(* Logix 5000 AddOnInstructionDefinition export Banner_K50ProL2_Param_v4; software revision 32.00 *)

TYPE Banner_IOL_Port_v4 :   // UDT that has all of the data items necessary to communicate with a specific Port on a IO-Link Master
STRUCT
   Port_Controlled : INT;   // Each bit represents a port on an IO-Link Master. Set to 1 to tell AOI to control that port.
   Port_Activate : INT;   // Each bit represents a port on an IO-Link Master. When ON that port will process any commands in queue.
   Port_Read : INT;   // Each bit represents a port on an IO-Link Master. Used to determine when device AOI has requested a Read command.
   Port_Write : INT;   // Each bit represents a port on an IO-Link Master. Used to determine when device AOI has requested a Write command.
   Port_RW_Complete : INT;   // Each bit represents a port on an IO-Link Master. Tells device AOI that Read or Write request has been completed.
   Port_Device_Read : INT;
   Data_Transfer : SINT[190];   // Array to transfer data from IO-Master to device AOIs.
END_STRUCT
END_TYPE

TYPE Banner_K50ProL2_CC_v2 :   // K50 Pro L2 Custom Color Setup Structure.
STRUCT
   Blue : INT;
   Green : INT;
   Red : INT;
   Color_Name : STRING;
END_STRUCT
END_TYPE

TYPE Banner_K50ProL2_RD_v2 :   // All of the read parameters for a K50 Pro L2
STRUCT
   Master_Cycle_Time : INT;
   Min_Cycle_Time : INT;
   M_Sequence_Capability : INT;
   IO_Link_Version_ID : INT;
   Process_Data_Input_Length : INT;
   Process_Data_Output_Length : INT;
   Combined_Vendor_ID : DINT;   // IO-Link Vendor ID
   Vendor_ID1 : INT;
   Vendor_ID2 : INT;
   Combined_Device_ID : DINT;   // IO-Link Device ID
   Device_ID1 : INT;
   Device_ID2 : INT;
   Device_ID3 : INT;
   Serial_Number : STRING;
END_STRUCT
END_TYPE

TYPE Banner_K50ProL2_v2 :   // All of the parameters for a K50 Pro L2.
STRUCT
   Initial_Global_Read : BOOL;   // Determines if all of the IO-Link data has been read into the PLC yet
   Command : INT;   // Value placed in here will activate a read or write to a specifc IO-Link Index
   Reset : BOOL;   // Resets AOI. This will force a complete parameter read of the sensor.
   Read_Data : Banner_K50ProL2_RD_v2;
   Write_Data : Banner_K50ProL2_WD_v2;
   Archive_Data : Banner_K50ProL2_WD_v2;
END_STRUCT
END_TYPE

TYPE Banner_K50ProL2_WD_v2 :   // All of the write parameters for a K50 Pro L2.
STRUCT
   System_Command : INT;
   Parameter_Access_Lock : SINT;
   Data_Storage_Lock : SINT;
   Local_Parameterization_Lock : SINT;
   Local_User_Interface_Lock : SINT;
   Reserved : INT;
   Restrict_To_Gamut : INT;
   Rotation_Speed : INT;
   Custom_Flash_Rate : INT;   // .5 to 20 Hz
   Custom_Intensity : INT;   // 0 to 100 = 0 to 100%
   Custom_Color : Banner_K50ProL2_CC_v2[6];
END_STRUCT
END_TYPE

ADD_ON_INSTRUCTION Banner_K50ProL2_Param_v4   (* revision 4.0, vendor Banner Engineering *)
// AOI to read and write parameter data to an IO-Link K50 Pro L2.
VAR_IN_OUT
   K50ProL2 : Banner_K50ProL2_v2; {required}
   Port_Data : Banner_IOL_Port_v4; {required}
END_VAR
VAR_INPUT
   Port : DINT; {required}
END_VAR
VAR
   Local_Control : DINT; {access None}
   Global_Read_Command_Value : INT; {access None}
   Global_Write_Command_Value : INT; {access None}
   Command_Being_Processed : BOOL; {access None}
   Index_Write_Inprocess : INT; {access None}
   Index_Write_Control : INT; {access None}
   Update_Archive : BOOL; {access None}
   Inprocess_Index : DINT; {access None}
   CC_R_Index : DINT; {access None}
   CC_WC_Index : DINT; {access None}
   CC_Index : DINT; {access None}
   CC_W_Index : DINT; {access None}
   CC_WC2_Index : DINT; {access None}
END_VAR

ROUTINE Logic   (* ladder *)
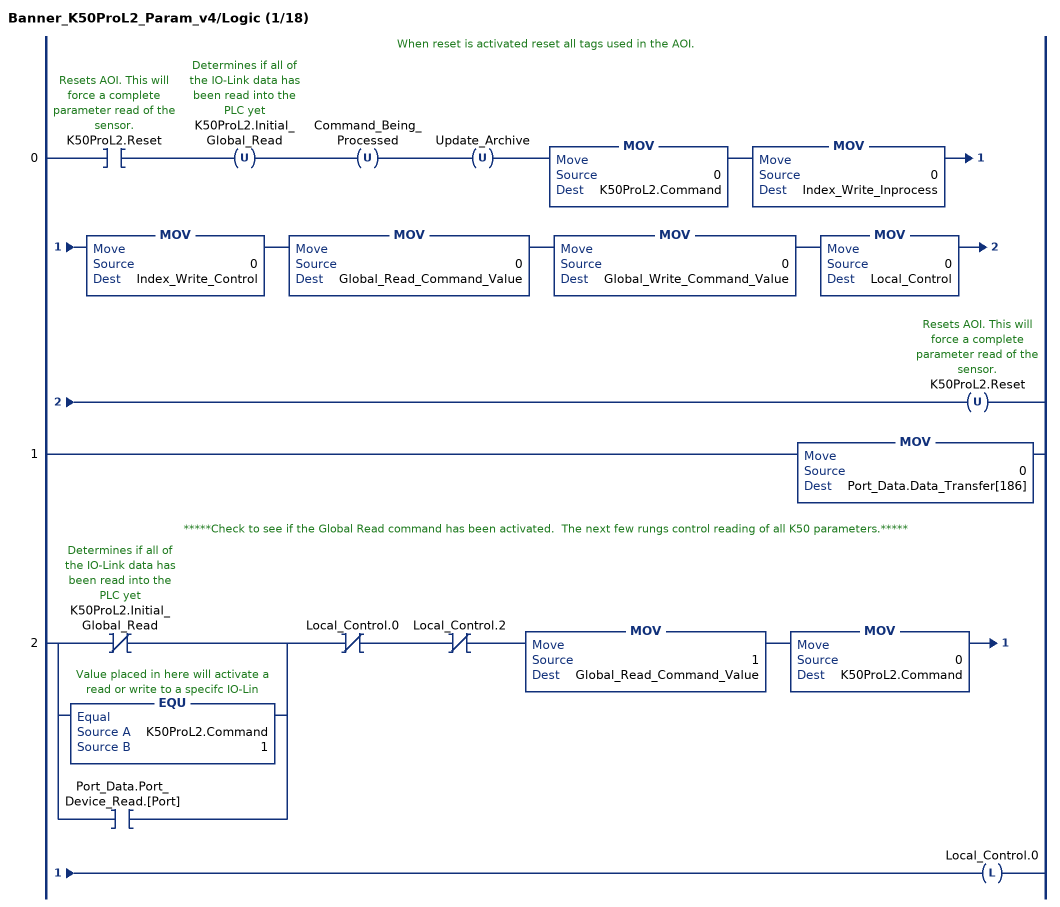
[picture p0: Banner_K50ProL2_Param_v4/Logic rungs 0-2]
   // When reset is activated reset all tags used in the AOI.
   0: XIC(K50ProL2.Reset)OTU(K50ProL2.Initial_Global_Read)OTU(Command_Being_Processed)OTU(Update_Archive)MOV(0,K50ProL2.Command)MOV(0,Index_Write_Inprocess)MOV(0,Index_Write_Control)MOV(0,Global_Read_Command_Value)MOV(0,Global_Write_Command_Value)MOV(0,Local_Control)OTU(K50ProL2.Reset);
   1: MOV(0,Port_Data.Data_Transfer[186]);
   // *****Check to see if the Global Read command has been activated.  The next few rungs control reading of all K50 parameters.*****
   2: [XIO(K50ProL2.Initial_Global_Read) ,EQU(K50ProL2.Command,1) ,XIC(Port_Data.Port_Device_Read.[Port]) ]XIO(Local_Control.0)XIO(Local_Control.2)MOV(1,Global_Read_Command_Value)MOV(0,K50ProL2.Command)OTL(Local_Control.0);
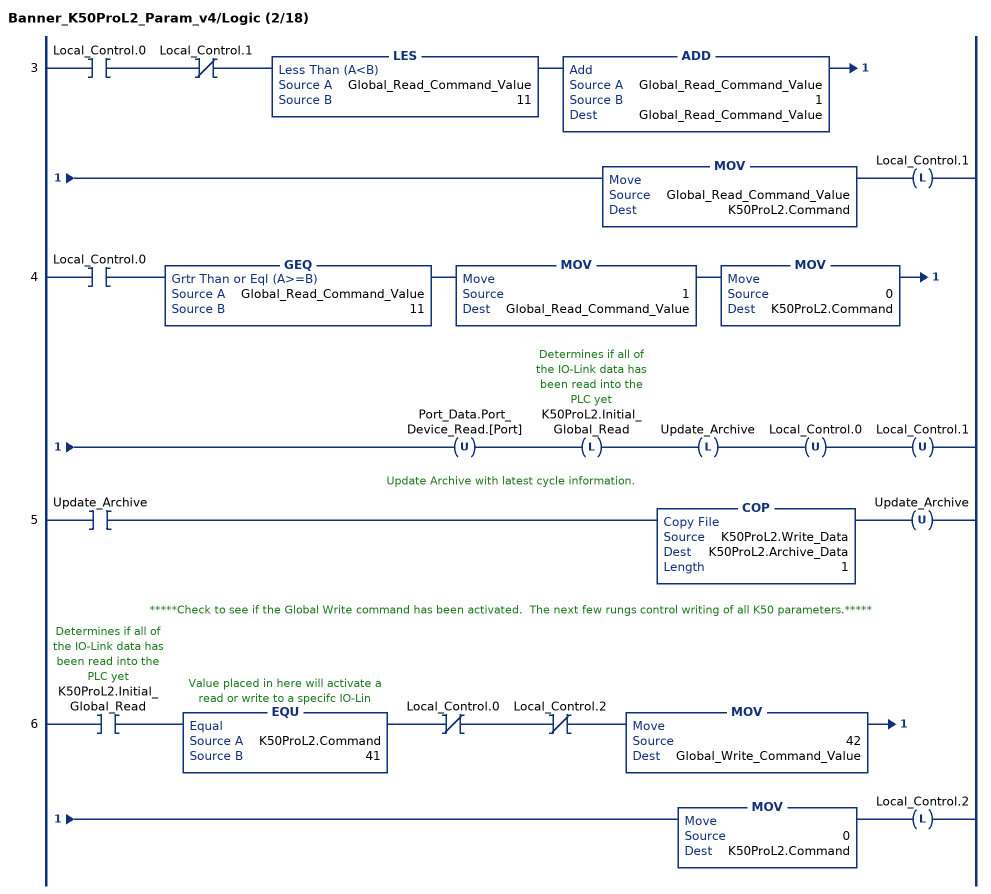
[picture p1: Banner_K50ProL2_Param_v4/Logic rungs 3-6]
   3: XIC(Local_Control.0)XIO(Local_Control.1)LES(Global_Read_Command_Value,11)ADD(Global_Read_Command_Value,1,Global_Read_Command_Value)MOV(Global_Read_Command_Value,K50ProL2.Command)OTL(Local_Control.1);
   4: XIC(Local_Control.0)GEQ(Global_Read_Command_Value,11)MOV(1,Global_Read_Command_Value)MOV(0,K50ProL2.Command)OTU(Port_Data.Port_Device_Read.[Port])OTL(K50ProL2.Initial_Global_Read)OTL(Update_Archive)OTU(Local_Control.0)OTU(Local_Control.1);
   // Update Archive with latest cycle information.
   5: XIC(Update_Archive)COP(K50ProL2.Write_Data,K50ProL2.Archive_Data,1)OTU(Update_Archive);
   // *****Check to see if the Global Write command has been activated.  The next few rungs control writing of all K50 parameters.*****
   6: XIC(K50ProL2.Initial_Global_Read)EQU(K50ProL2.Command,41)XIO(Local_Control.0)XIO(Local_Control.2)MOV(42,Global_Write_Command_Value)MOV(0,K50ProL2.Command)OTL(Local_Control.2);
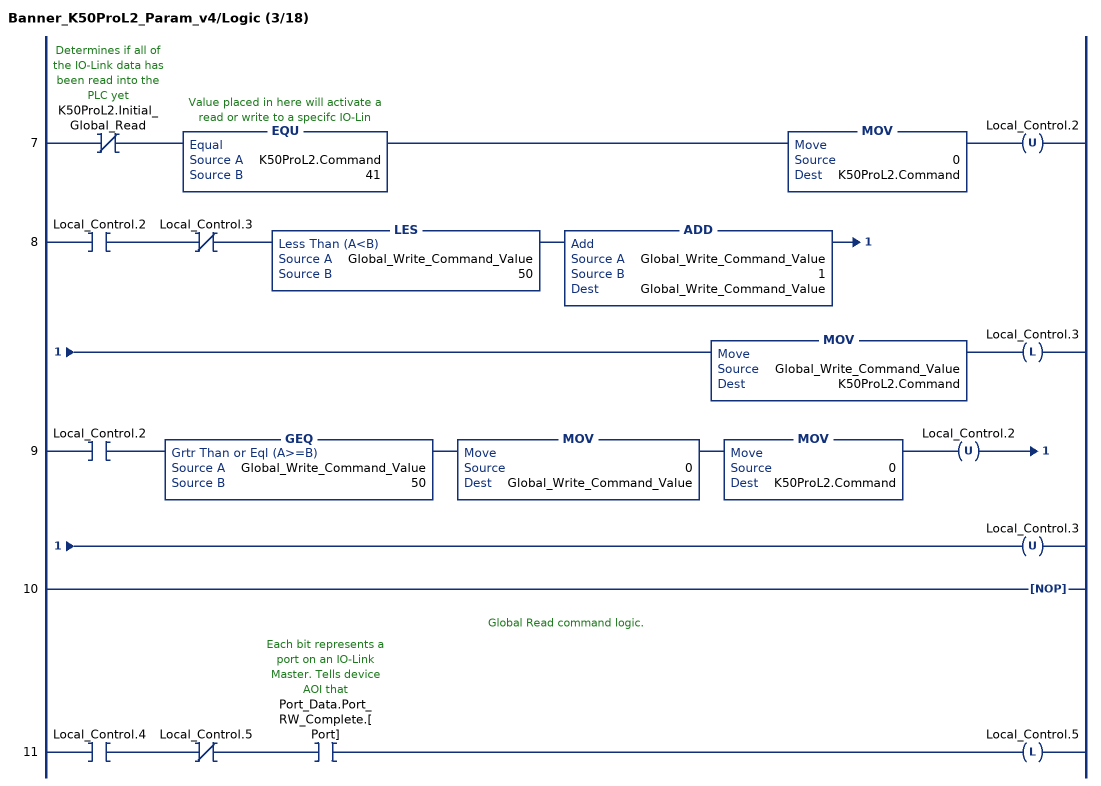
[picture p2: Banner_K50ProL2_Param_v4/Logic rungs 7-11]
   7: XIO(K50ProL2.Initial_Global_Read)EQU(K50ProL2.Command,41)MOV(0,K50ProL2.Command)OTU(Local_Control.2);
   8: XIC(Local_Control.2)XIO(Local_Control.3)LES(Global_Write_Command_Value,50)ADD(Global_Write_Command_Value,1,Global_Write_Command_Value)MOV(Global_Write_Command_Value,K50ProL2.Command)OTL(Local_Control.3);
   9: XIC(Local_Control.2)GEQ(Global_Write_Command_Value,50)MOV(0,Global_Write_Command_Value)MOV(0,K50ProL2.Command)OTU(Local_Control.2)OTU(Local_Control.3);
   10: NOP();
   // Global Read command logic.
   11: XIC(Local_Control.4)XIO(Local_Control.5)XIC(Port_Data.Port_RW_Complete.[Port])OTL(Local_Control.5);
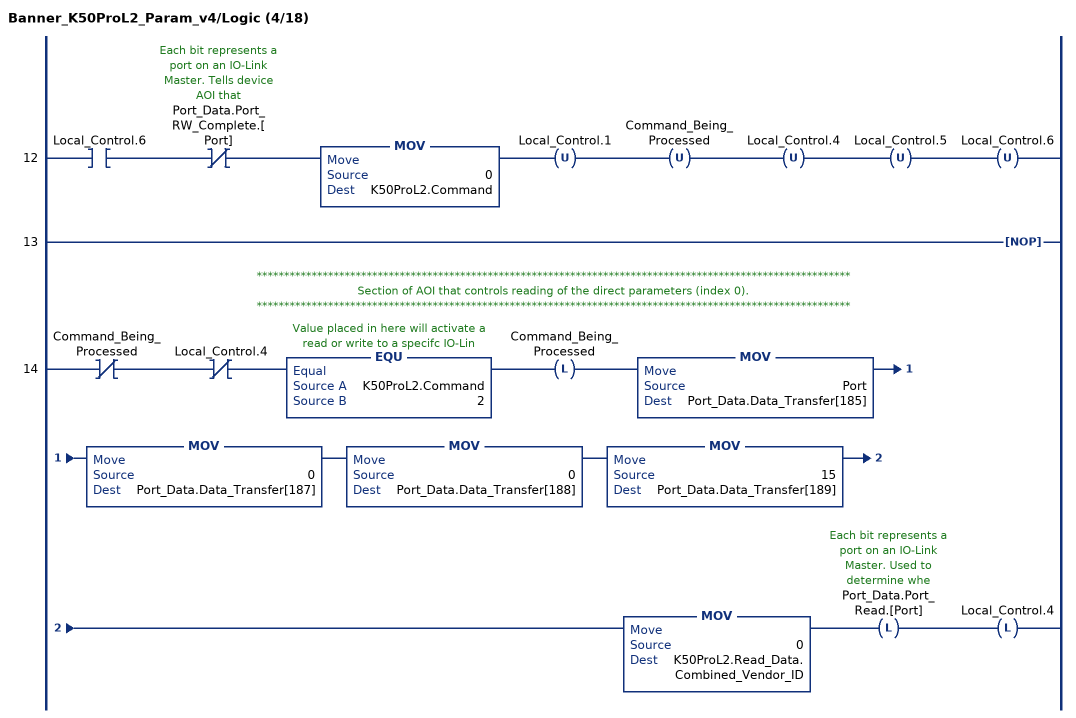
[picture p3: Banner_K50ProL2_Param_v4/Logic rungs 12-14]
   12: XIC(Local_Control.6)XIO(Port_Data.Port_RW_Complete.[Port])MOV(0,K50ProL2.Command)OTU(Local_Control.1)OTU(Command_Being_Processed)OTU(Local_Control.4)OTU(Local_Control.5)OTU(Local_Control.6);
   13: NOP();
   // ************************************************************************************************************
   // Section of AOI that controls reading of the direct parameters (index 0).
   // ************************************************************************************************************
   14: XIO(Command_Being_Processed)XIO(Local_Control.4)EQU(K50ProL2.Command,2)OTL(Command_Being_Processed)MOV(Port,Port_Data.Data_Transfer[185])MOV(0,Port_Data.Data_Transfer[187])MOV(0,Port_Data.Data_Transfer[188])MOV(15,Port_Data.Data_Transfer[189])MOV(0,K50ProL2.Read_Data.Combined_Vendor_ID)OTL(Port_Data.Port_Read.[Port])OTL(Local_Control.4);
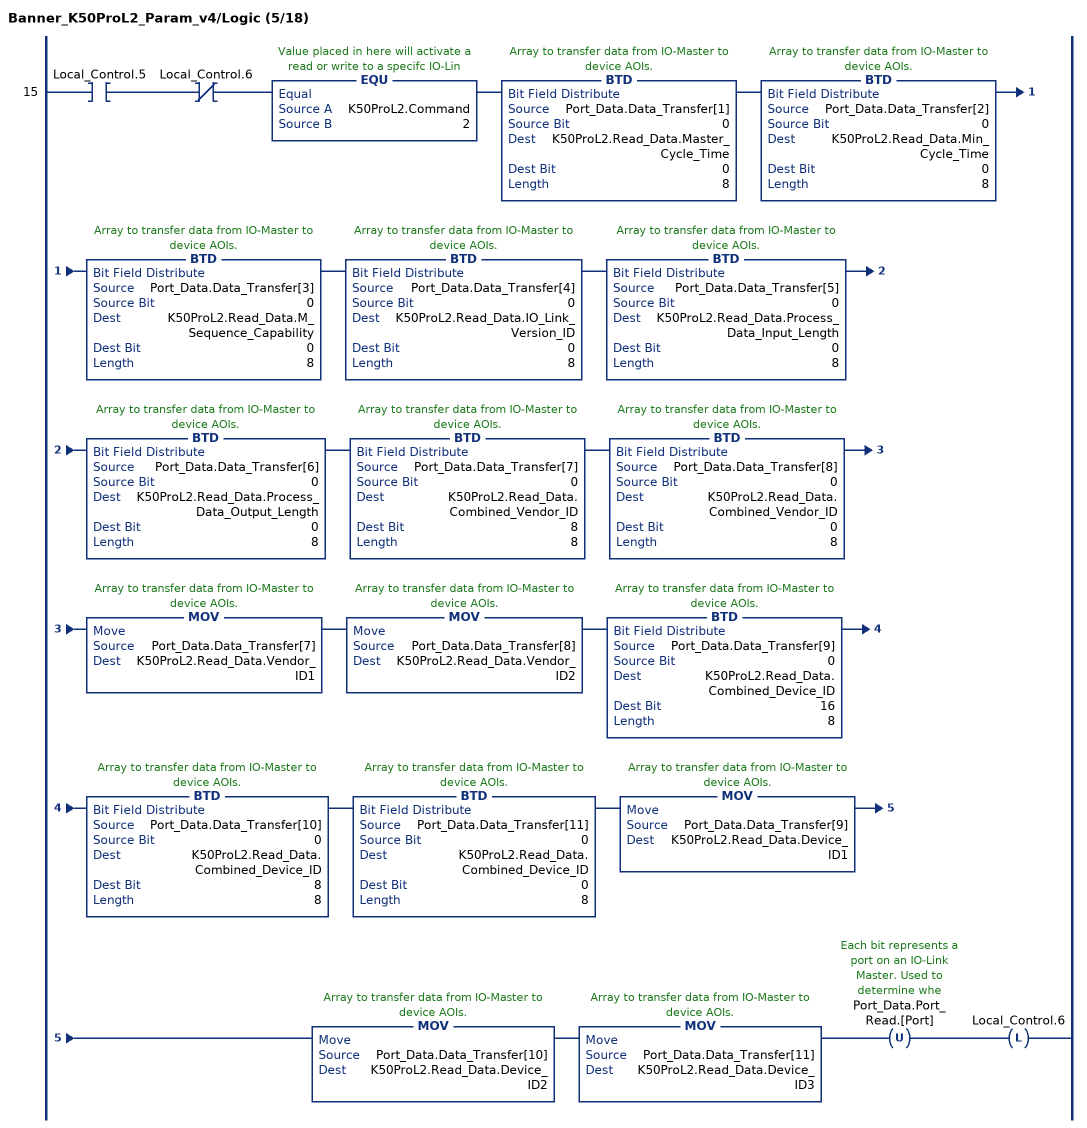
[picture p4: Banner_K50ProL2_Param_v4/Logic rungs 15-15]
   15: XIC(Local_Control.5)XIO(Local_Control.6)EQU(K50ProL2.Command,2)BTD(Port_Data.Data_Transfer[1],0,K50ProL2.Read_Data.Master_Cycle_Time,0,8)BTD(Port_Data.Data_Transfer[2],0,K50ProL2.Read_Data.Min_Cycle_Time,0,8)BTD(Port_Data.Data_Transfer[3],0,K50ProL2.Read_Data.M_Sequence_Capability,0,8)BTD(Port_Data.Data_Transfer[4],0,K50ProL2.Read_Data.IO_Link_Version_ID,0,8)BTD(Port_Data.Data_Transfer[5],0,K50ProL2.Read_Data.Process_Data_Input_Length,0,8)BTD(Port_Data.Data_Transfer[6],0,K50ProL2.Read_Data.Process_Data_Output_Length,0,8)BTD(Port_Data.Data_Transfer[7],0,K50ProL2.Read_Data.Combined_Vendor_ID,8,8)BTD(Port_Data.Data_Transfer[8],0,K50ProL2.Read_Data.Combined_Vendor_ID,0,8)MOV(Port_Data.Data_Transfer[7],K50ProL2.Read_Data.Vendor_ID1)MOV(Port_Data.Data_Transfer[8],K50ProL2.Read_Data.Vendor_ID2)BTD(Port_Data.Data_Transfer[9],0,K50ProL2.Read_Data.Combined_Device_ID,16,8)BTD(Port_Data.Data_Transfer[10],0,K50ProL2.Read_Data.Combined_Device_ID,8,8)BTD(Port_Data.Data_Transfer[11],0,K50ProL2.Read_Data.Combined_Device_ID,0,8)MOV(Port_Data.Data_Transfer[9],K50ProL2.Read_Data.Device_ID1)MOV(Port_Data.Data_Transfer[10],K50ProL2.Read_Data.Device_ID2)MOV(Port_Data.Data_Transfer[11],K50ProL2.Read_Data.Device_ID3)OTU(Port_Data.Port_Read.[Port])OTL(Local_Control.6);
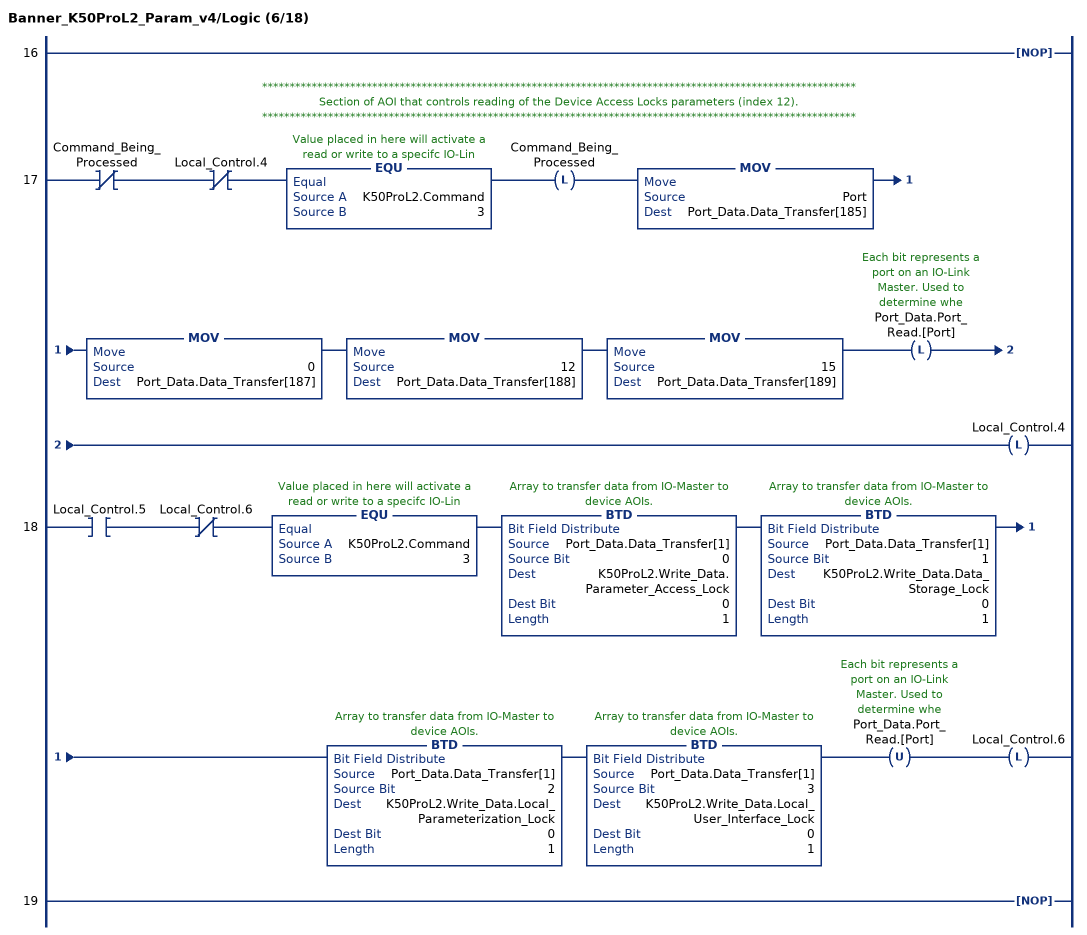
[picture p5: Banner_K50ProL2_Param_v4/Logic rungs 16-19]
   16: NOP();
   // ************************************************************************************************************
   // Section of AOI that controls reading of the Device Access Locks parameters (index 12).
   // ************************************************************************************************************
   17: XIO(Command_Being_Processed)XIO(Local_Control.4)EQU(K50ProL2.Command,3)OTL(Command_Being_Processed)MOV(Port,Port_Data.Data_Transfer[185])MOV(0,Port_Data.Data_Transfer[187])MOV(12,Port_Data.Data_Transfer[188])MOV(15,Port_Data.Data_Transfer[189])OTL(Port_Data.Port_Read.[Port])OTL(Local_Control.4);
   18: XIC(Local_Control.5)XIO(Local_Control.6)EQU(K50ProL2.Command,3)BTD(Port_Data.Data_Transfer[1],0,K50ProL2.Write_Data.Parameter_Access_Lock,0,1)BTD(Port_Data.Data_Transfer[1],1,K50ProL2.Write_Data.Data_Storage_Lock,0,1)BTD(Port_Data.Data_Transfer[1],2,K50ProL2.Write_Data.Local_Parameterization_Lock,0,1)BTD(Port_Data.Data_Transfer[1],3,K50ProL2.Write_Data.Local_User_Interface_Lock,0,1)OTU(Port_Data.Port_Read.[Port])OTL(Local_Control.6);
   19: NOP();
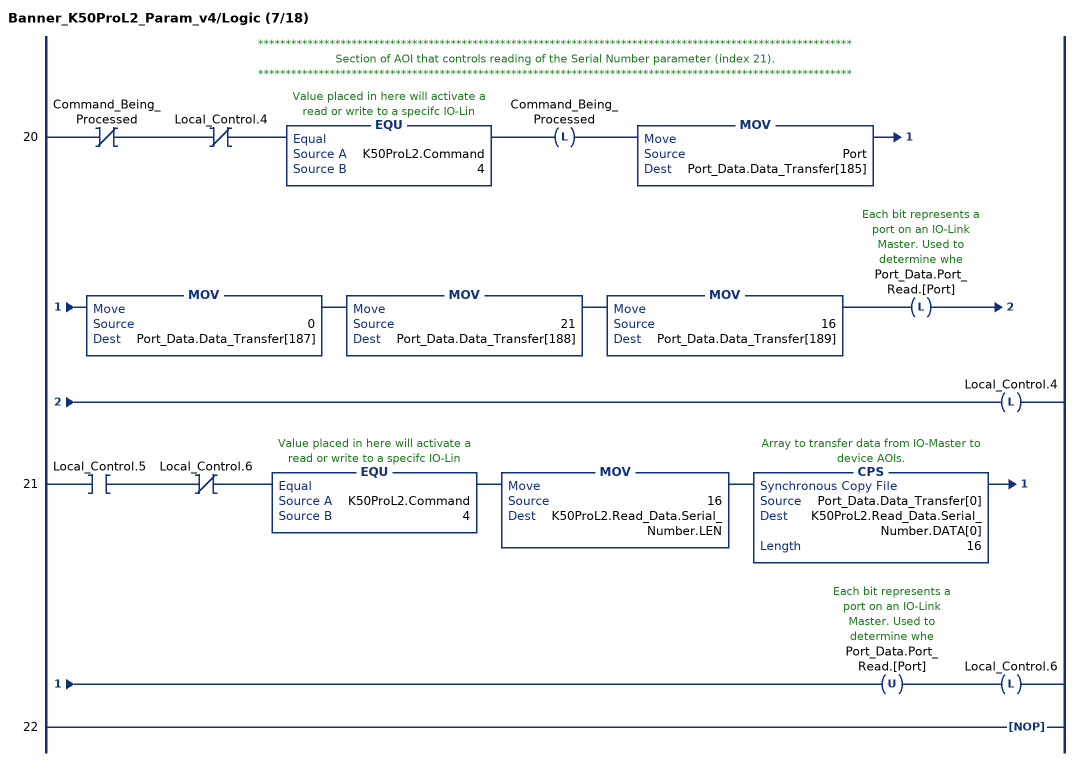
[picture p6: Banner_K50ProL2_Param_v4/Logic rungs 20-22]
   // ************************************************************************************************************
   // Section of AOI that controls reading of the Serial Number parameter (index 21).
   // ************************************************************************************************************
   20: XIO(Command_Being_Processed)XIO(Local_Control.4)EQU(K50ProL2.Command,4)OTL(Command_Being_Processed)MOV(Port,Port_Data.Data_Transfer[185])MOV(0,Port_Data.Data_Transfer[187])MOV(21,Port_Data.Data_Transfer[188])MOV(16,Port_Data.Data_Transfer[189])OTL(Port_Data.Port_Read.[Port])OTL(Local_Control.4);
   21: XIC(Local_Control.5)XIO(Local_Control.6)EQU(K50ProL2.Command,4)MOV(16,K50ProL2.Read_Data.Serial_Number.LEN)CPS(Port_Data.Data_Transfer[0],K50ProL2.Read_Data.Serial_Number.DATA[0],16)OTU(Port_Data.Port_Read.[Port])OTL(Local_Control.6);
   22: NOP();
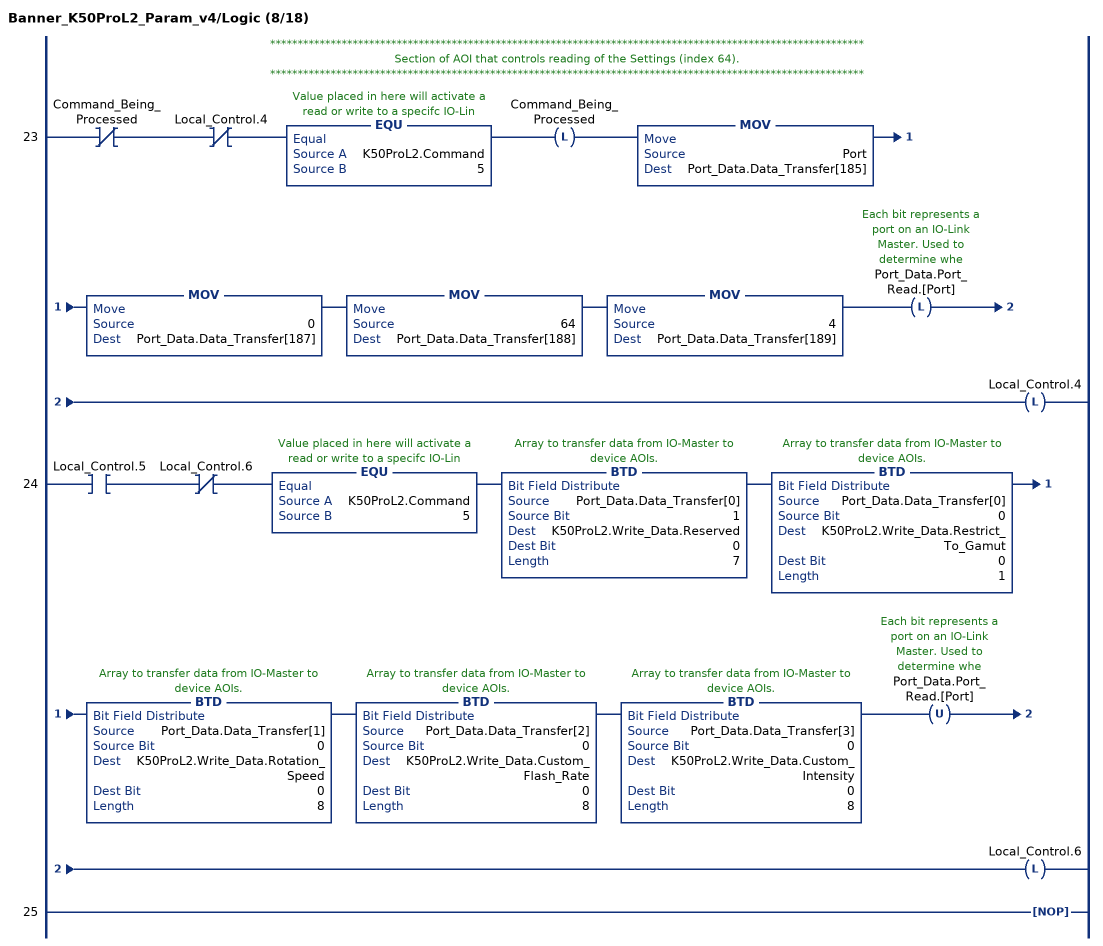
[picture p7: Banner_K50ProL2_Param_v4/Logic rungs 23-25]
   // ************************************************************************************************************
   // Section of AOI that controls reading of the Settings (index 64).
   // ************************************************************************************************************
   23: XIO(Command_Being_Processed)XIO(Local_Control.4)EQU(K50ProL2.Command,5)OTL(Command_Being_Processed)MOV(Port,Port_Data.Data_Transfer[185])MOV(0,Port_Data.Data_Transfer[187])MOV(64,Port_Data.Data_Transfer[188])MOV(4,Port_Data.Data_Transfer[189])OTL(Port_Data.Port_Read.[Port])OTL(Local_Control.4);
   24: XIC(Local_Control.5)XIO(Local_Control.6)EQU(K50ProL2.Command,5)BTD(Port_Data.Data_Transfer[0],1,K50ProL2.Write_Data.Reserved,0,7)BTD(Port_Data.Data_Transfer[0],0,K50ProL2.Write_Data.Restrict_To_Gamut,0,1)BTD(Port_Data.Data_Transfer[1],0,K50ProL2.Write_Data.Rotation_Speed,0,8)BTD(Port_Data.Data_Transfer[2],0,K50ProL2.Write_Data.Custom_Flash_Rate,0,8)BTD(Port_Data.Data_Transfer[3],0,K50ProL2.Write_Data.Custom_Intensity,0,8)OTU(Port_Data.Port_Read.[Port])OTL(Local_Control.6);
   25: NOP();
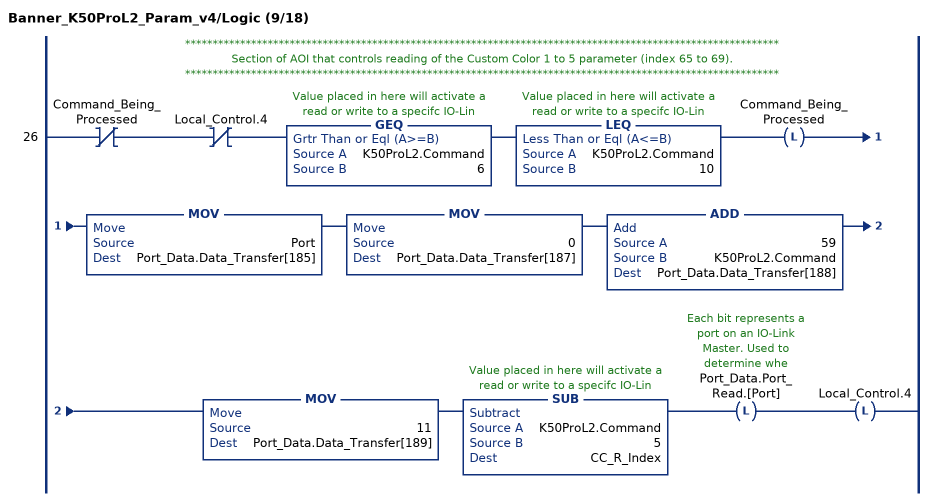
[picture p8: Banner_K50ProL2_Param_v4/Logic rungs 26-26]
   // ************************************************************************************************************
   // Section of AOI that controls reading of the Custom Color 1 to 5 parameter (index 65 to 69).
   // ************************************************************************************************************
   26: XIO(Command_Being_Processed)XIO(Local_Control.4)GEQ(K50ProL2.Command,6)LEQ(K50ProL2.Command,10)OTL(Command_Being_Processed)MOV(Port,Port_Data.Data_Transfer[185])MOV(0,Port_Data.Data_Transfer[187])ADD(59,K50ProL2.Command,Port_Data.Data_Transfer[188])MOV(11,Port_Data.Data_Transfer[189])SUB(K50ProL2.Command,5,CC_R_Index)OTL(Port_Data.Port_Read.[Port])OTL(Local_Control.4);
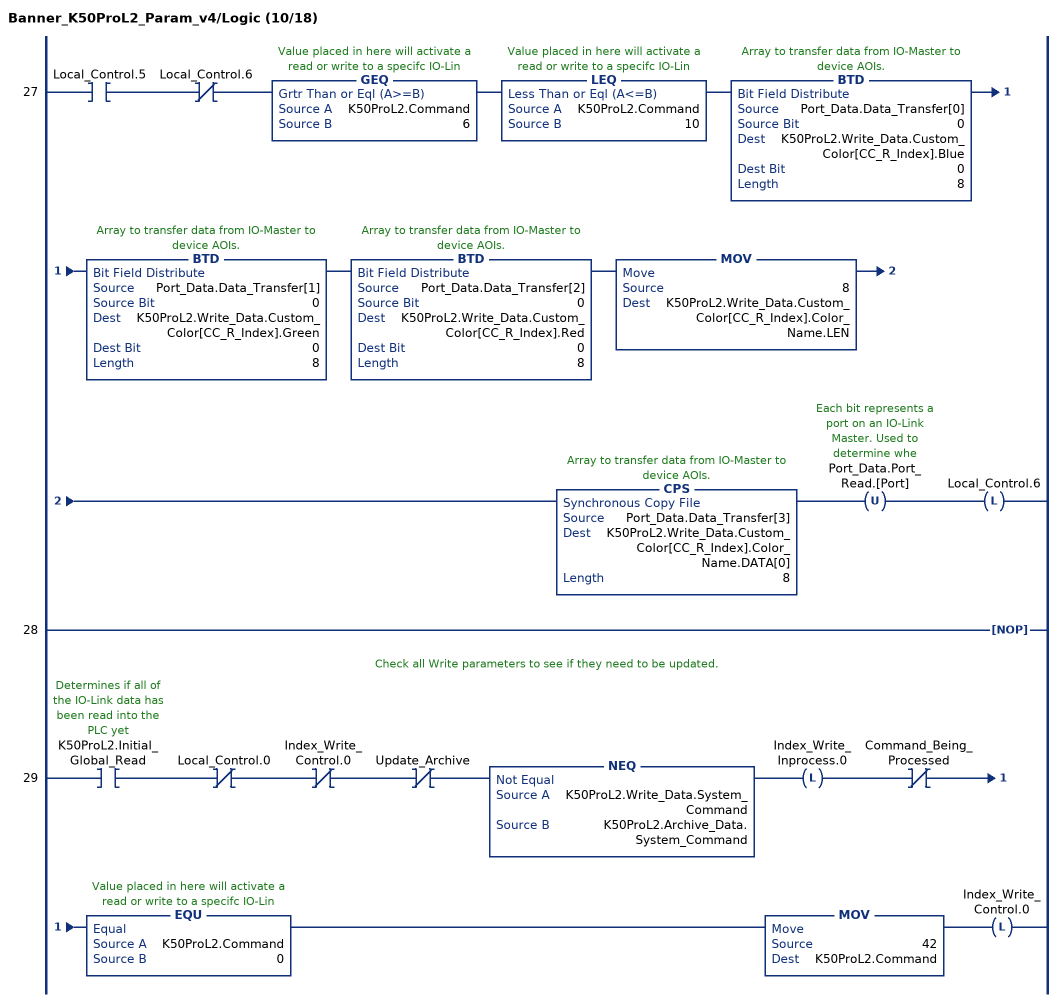
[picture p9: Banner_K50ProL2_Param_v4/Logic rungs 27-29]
   27: XIC(Local_Control.5)XIO(Local_Control.6)GEQ(K50ProL2.Command,6)LEQ(K50ProL2.Command,10)BTD(Port_Data.Data_Transfer[0],0,K50ProL2.Write_Data.Custom_Color[CC_R_Index].Blue,0,8)BTD(Port_Data.Data_Transfer[1],0,K50ProL2.Write_Data.Custom_Color[CC_R_Index].Green,0,8)BTD(Port_Data.Data_Transfer[2],0,K50ProL2.Write_Data.Custom_Color[CC_R_Index].Red,0,8)MOV(8,K50ProL2.Write_Data.Custom_Color[CC_R_Index].Color_Name.LEN)CPS(Port_Data.Data_Transfer[3],K50ProL2.Write_Data.Custom_Color[CC_R_Index].Color_Name.DATA[0],8)OTU(Port_Data.Port_Read.[Port])OTL(Local_Control.6);
   28: NOP();
   // Check all Write parameters to see if they need to be updated.
   29: XIC(K50ProL2.Initial_Global_Read)XIO(Local_Control.0)XIO(Index_Write_Control.0)XIO(Update_Archive)NEQ(K50ProL2.Write_Data.System_Command,K50ProL2.Archive_Data.System_Command)OTL(Index_Write_Inprocess.0)XIO(Command_Being_Processed)EQU(K50ProL2.Command,0)MOV(42,K50ProL2.Command)OTL(Index_Write_Control.0);
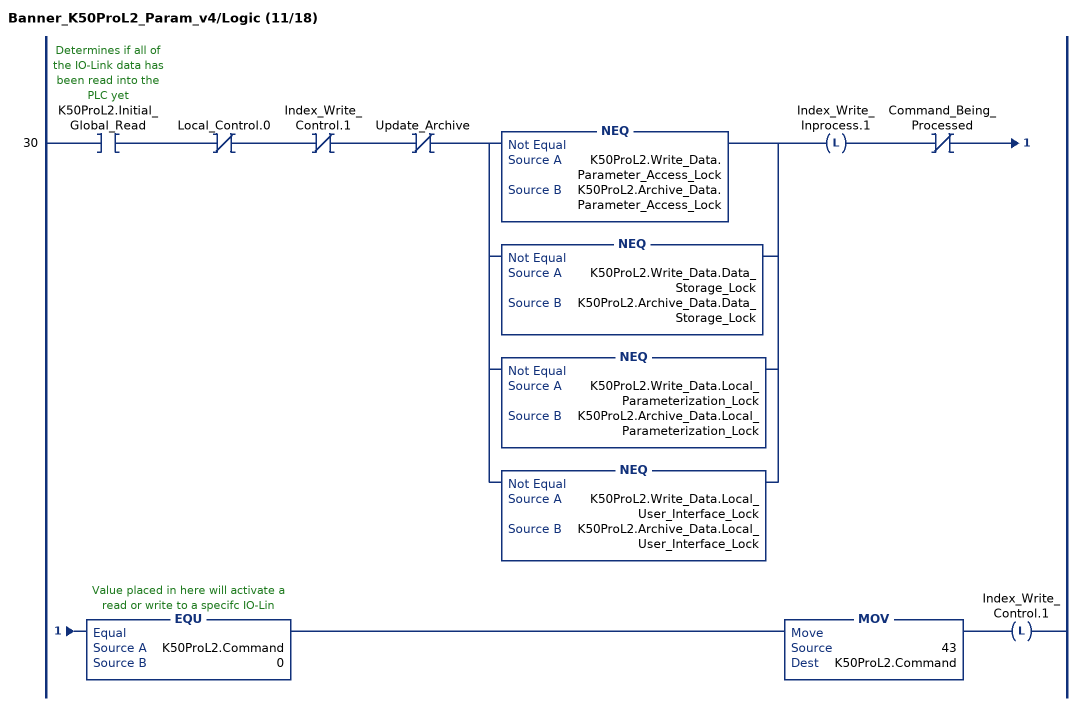
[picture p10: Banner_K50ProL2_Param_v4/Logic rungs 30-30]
   30: XIC(K50ProL2.Initial_Global_Read)XIO(Local_Control.0)XIO(Index_Write_Control.1)XIO(Update_Archive)[NEQ(K50ProL2.Write_Data.Parameter_Access_Lock,K50ProL2.Archive_Data.Parameter_Access_Lock) ,NEQ(K50ProL2.Write_Data.Data_Storage_Lock,K50ProL2.Archive_Data.Data_Storage_Lock) ,NEQ(K50ProL2.Write_Data.Local_Parameterization_Lock,K50ProL2.Archive_Data.Local_Parameterization_Lock) ,NEQ(K50ProL2.Write_Data.Local_User_Interface_Lock,K50ProL2.Archive_Data.Local_User_Interface_Lock) ]OTL(Index_Write_Inprocess.1)XIO(Command_Being_Processed)EQU(K50ProL2.Command,0)MOV(43,K50ProL2.Command)OTL(Index_Write_Control.1);
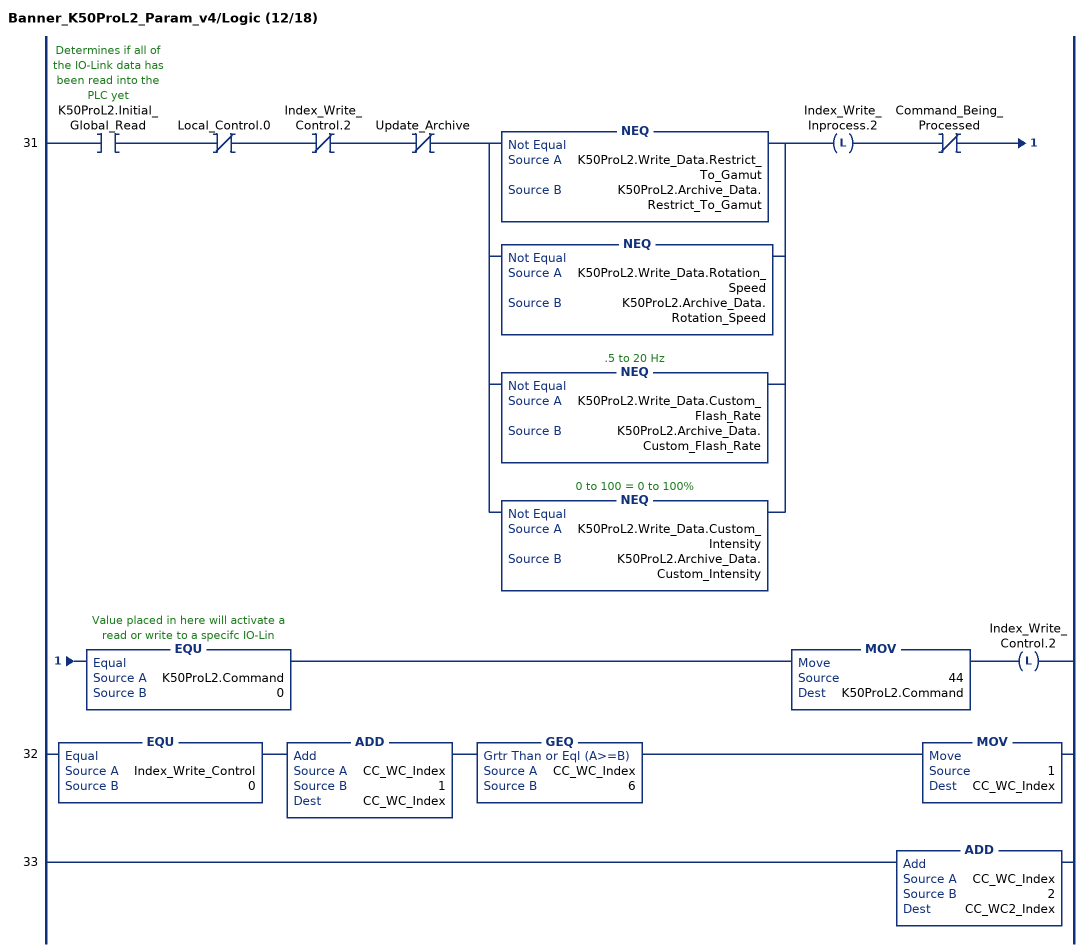
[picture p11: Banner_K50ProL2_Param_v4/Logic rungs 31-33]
   31: XIC(K50ProL2.Initial_Global_Read)XIO(Local_Control.0)XIO(Index_Write_Control.2)XIO(Update_Archive)[NEQ(K50ProL2.Write_Data.Restrict_To_Gamut,K50ProL2.Archive_Data.Restrict_To_Gamut) ,NEQ(K50ProL2.Write_Data.Rotation_Speed,K50ProL2.Archive_Data.Rotation_Speed) ,NEQ(K50ProL2.Write_Data.Custom_Flash_Rate,K50ProL2.Archive_Data.Custom_Flash_Rate) ,NEQ(K50ProL2.Write_Data.Custom_Intensity,K50ProL2.Archive_Data.Custom_Intensity) ]OTL(Index_Write_Inprocess.2)XIO(Command_Being_Processed)EQU(K50ProL2.Command,0)MOV(44,K50ProL2.Command)OTL(Index_Write_Control.2);
   32: EQU(Index_Write_Control,0)ADD(CC_WC_Index,1,CC_WC_Index)GEQ(CC_WC_Index,6)MOV(1,CC_WC_Index);
   33: ADD(CC_WC_Index,2,CC_WC2_Index);
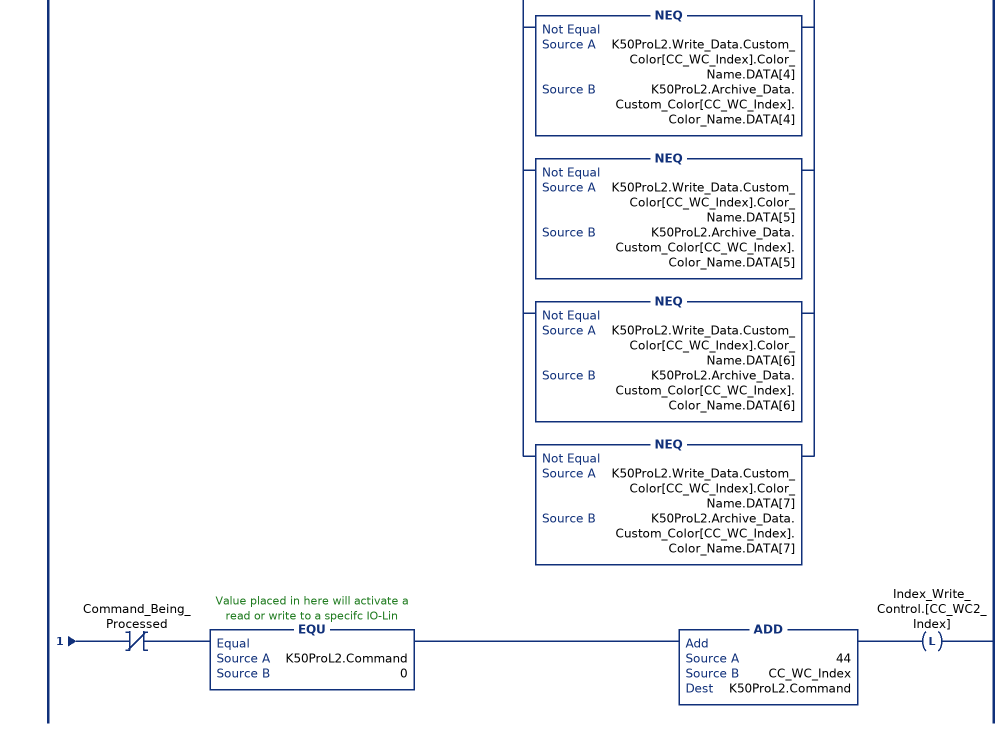
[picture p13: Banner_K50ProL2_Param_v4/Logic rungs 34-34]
   34: XIC(K50ProL2.Initial_Global_Read)XIO(Local_Control.0)XIO(Index_Write_Control.[CC_WC2_Index])XIO(Update_Archive)[NEQ(K50ProL2.Write_Data.Custom_Color[CC_WC_Index].Blue,K50ProL2.Archive_Data.Custom_Color[CC_WC_Index].Blue) ,NEQ(K50ProL2.Write_Data.Custom_Color[CC_WC_Index].Green,K50ProL2.Archive_Data.Custom_Color[CC_WC_Index].Green) ,NEQ(K50ProL2.Write_Data.Custom_Color[CC_WC_Index].Red,K50ProL2.Archive_Data.Custom_Color[CC_WC_Index].Red) ,NEQ(K50ProL2.Write_Data.Custom_Color[CC_WC_Index].Color_Name.DATA[0],K50ProL2.Archive_Data.Custom_Color[CC_WC_Index].Color_Name.DATA[0]) ,NEQ(K50ProL2.Write_Data.Custom_Color[CC_WC_Index].Color_Name.DATA[1],K50ProL2.Archive_Data.Custom_Color[CC_WC_Index].Color_Name.DATA[1]) ,NEQ(K50ProL2.Write_Data.Custom_Color[CC_WC_Index].Color_Name.DATA[2],K50ProL2.Archive_Data.Custom_Color[CC_WC_Index].Color_Name.DATA[2]) ,NEQ(K50ProL2.Write_Data.Custom_Color[CC_WC_Index].Color_Name.DATA[3],K50ProL2.Archive_Data.Custom_Color[CC_WC_Index].Color_Name.DATA[3]) ,NEQ(K50ProL2.Write_Data.Custom_Color[CC_WC_Index].Color_Name.DATA[4],K50ProL2.Archive_Data.Custom_Color[CC_WC_Index].Color_Name.DATA[4]) ,NEQ(K50ProL2.Write_Data.Custom_Color[CC_WC_Index].Color_Name.DATA[5],K50ProL2.Archive_Data.Custom_Color[CC_WC_Index].Color_Name.DATA[5]) ,NEQ(K50ProL2.Write_Data.Custom_Color[CC_WC_Index].Color_Name.DATA[6],K50ProL2.Archive_Data.Custom_Color[CC_WC_Index].Color_Name.DATA[6]) ,NEQ(K50ProL2.Write_Data.Custom_Color[CC_WC_Index].Color_Name.DATA[7],K50ProL2.Archive_Data.Custom_Color[CC_WC_Index].Color_Name.DATA[7]) ]OTL(Index_Write_Inprocess.[CC_WC2_Index])XIO(Command_Being_Processed)EQU(K50ProL2.Command,0)ADD(44,CC_WC_Index,K50ProL2.Command)OTL(Index_Write_Control.[CC_WC2_Index]);
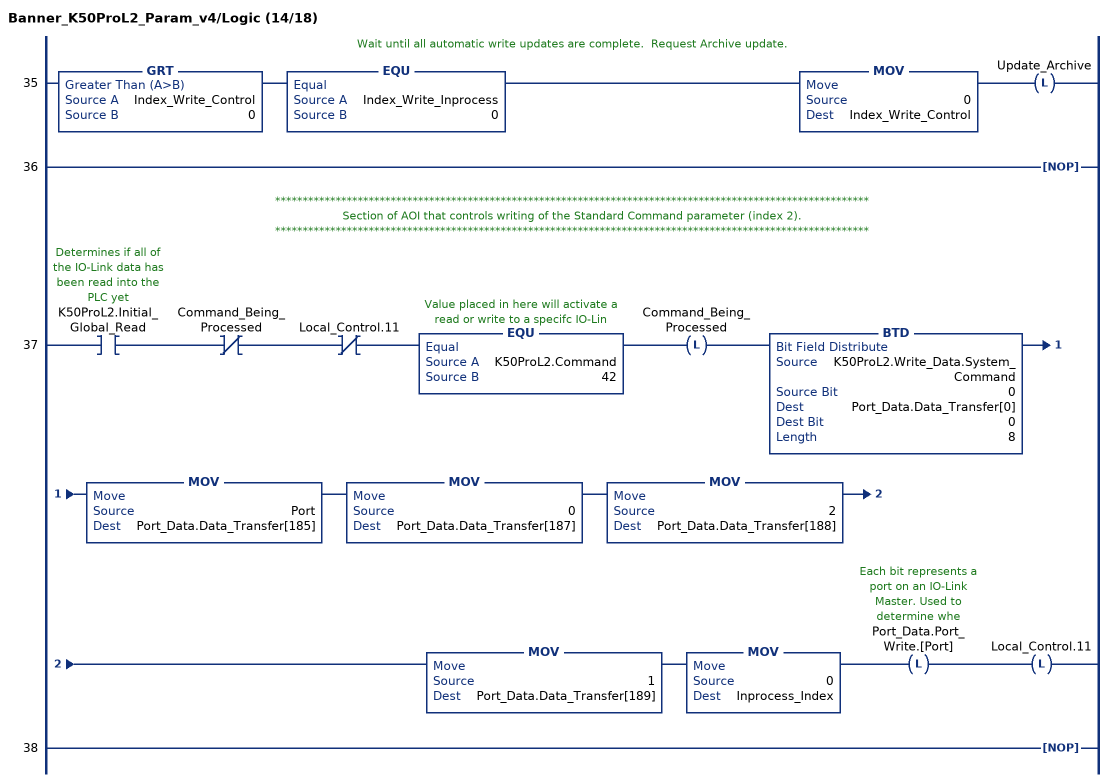
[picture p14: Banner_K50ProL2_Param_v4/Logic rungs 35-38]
   // Wait until all automatic write updates are complete.  Request Archive update.
   35: GRT(Index_Write_Control,0)EQU(Index_Write_Inprocess,0)MOV(0,Index_Write_Control)OTL(Update_Archive);
   36: NOP();
   // ************************************************************************************************************
   // Section of AOI that controls writing of the Standard Command parameter (index 2).
   // ************************************************************************************************************
   37: XIC(K50ProL2.Initial_Global_Read)XIO(Command_Being_Processed)XIO(Local_Control.11)EQU(K50ProL2.Command,42)OTL(Command_Being_Processed)BTD(K50ProL2.Write_Data.System_Command,0,Port_Data.Data_Transfer[0],0,8)MOV(Port,Port_Data.Data_Transfer[185])MOV(0,Port_Data.Data_Transfer[187])MOV(2,Port_Data.Data_Transfer[188])MOV(1,Port_Data.Data_Transfer[189])MOV(0,Inprocess_Index)OTL(Port_Data.Port_Write.[Port])OTL(Local_Control.11);
   38: NOP();
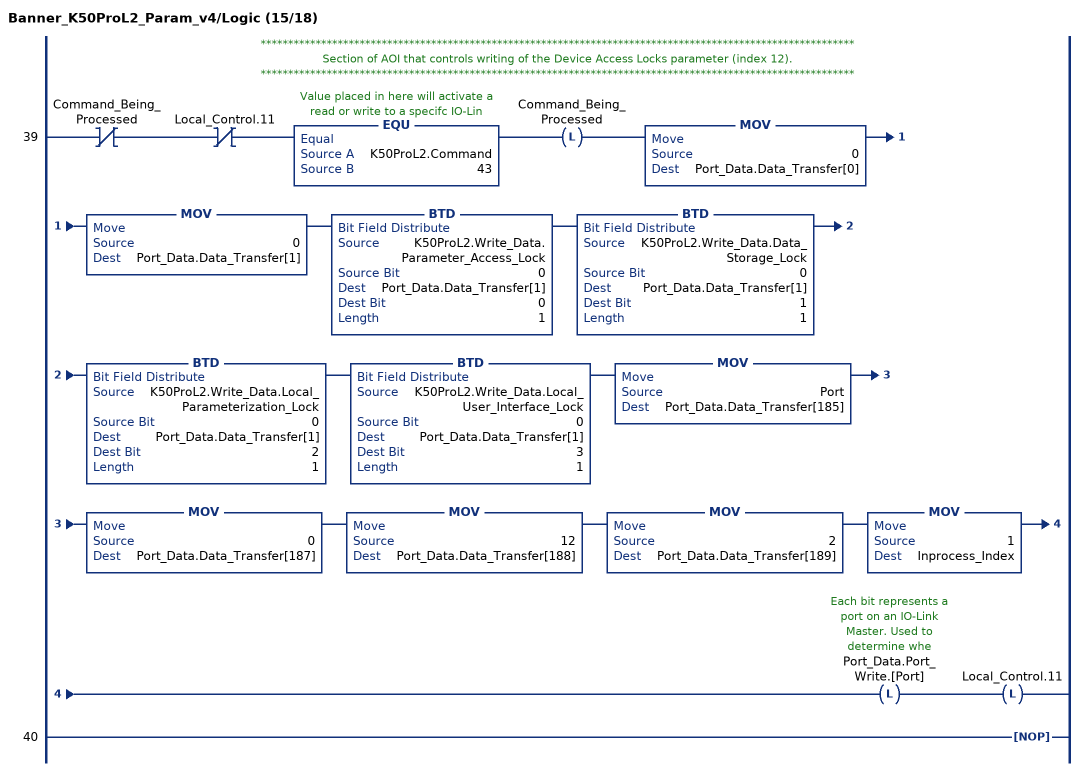
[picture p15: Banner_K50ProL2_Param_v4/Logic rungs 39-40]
   // ************************************************************************************************************
   // Section of AOI that controls writing of the Device Access Locks parameter (index 12).
   // ************************************************************************************************************
   39: XIO(Command_Being_Processed)XIO(Local_Control.11)EQU(K50ProL2.Command,43)OTL(Command_Being_Processed)MOV(0,Port_Data.Data_Transfer[0])MOV(0,Port_Data.Data_Transfer[1])BTD(K50ProL2.Write_Data.Parameter_Access_Lock,0,Port_Data.Data_Transfer[1],0,1)BTD(K50ProL2.Write_Data.Data_Storage_Lock,0,Port_Data.Data_Transfer[1],1,1)BTD(K50ProL2.Write_Data.Local_Parameterization_Lock,0,Port_Data.Data_Transfer[1],2,1)BTD(K50ProL2.Write_Data.Local_User_Interface_Lock,0,Port_Data.Data_Transfer[1],3,1)MOV(Port,Port_Data.Data_Transfer[185])MOV(0,Port_Data.Data_Transfer[187])MOV(12,Port_Data.Data_Transfer[188])MOV(2,Port_Data.Data_Transfer[189])MOV(1,Inprocess_Index)OTL(Port_Data.Port_Write.[Port])OTL(Local_Control.11);
   40: NOP();
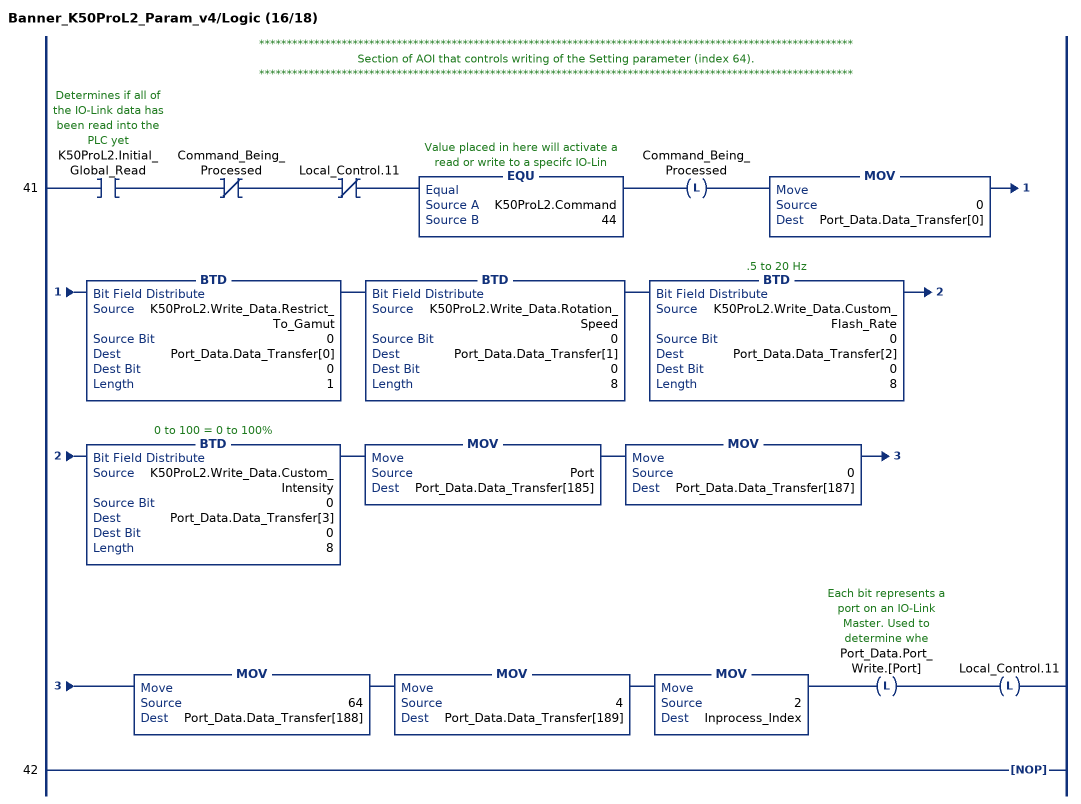
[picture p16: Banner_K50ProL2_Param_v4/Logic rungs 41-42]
   // ************************************************************************************************************
   // Section of AOI that controls writing of the Setting parameter (index 64).
   // ************************************************************************************************************
   41: XIC(K50ProL2.Initial_Global_Read)XIO(Command_Being_Processed)XIO(Local_Control.11)EQU(K50ProL2.Command,44)OTL(Command_Being_Processed)MOV(0,Port_Data.Data_Transfer[0])BTD(K50ProL2.Write_Data.Restrict_To_Gamut,0,Port_Data.Data_Transfer[0],0,1)BTD(K50ProL2.Write_Data.Rotation_Speed,0,Port_Data.Data_Transfer[1],0,8)BTD(K50ProL2.Write_Data.Custom_Flash_Rate,0,Port_Data.Data_Transfer[2],0,8)BTD(K50ProL2.Write_Data.Custom_Intensity,0,Port_Data.Data_Transfer[3],0,8)MOV(Port,Port_Data.Data_Transfer[185])MOV(0,Port_Data.Data_Transfer[187])MOV(64,Port_Data.Data_Transfer[188])MOV(4,Port_Data.Data_Transfer[189])MOV(2,Inprocess_Index)OTL(Port_Data.Port_Write.[Port])OTL(Local_Control.11);
   42: NOP();
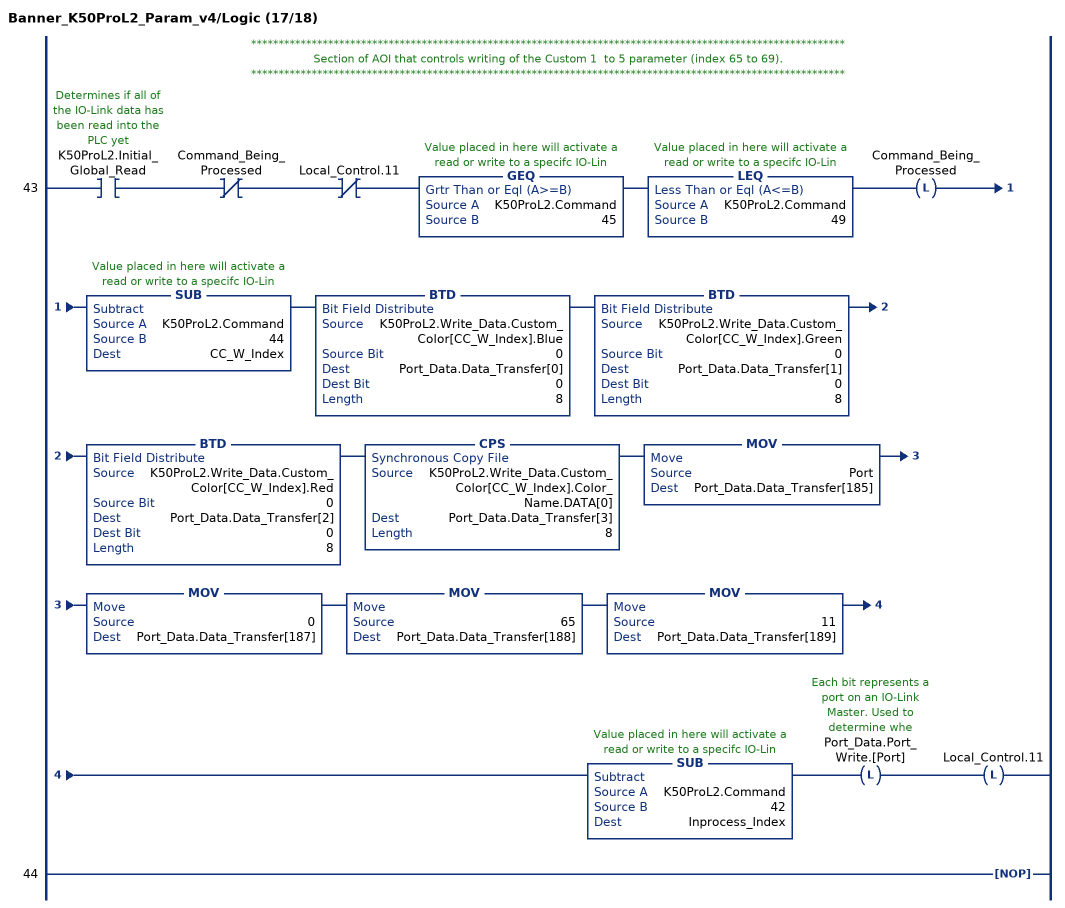
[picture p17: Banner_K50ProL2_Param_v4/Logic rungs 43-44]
   // ************************************************************************************************************
   // Section of AOI that controls writing of the Custom 1  to 5 parameter (index 65 to 69).
   // ************************************************************************************************************
   43: XIC(K50ProL2.Initial_Global_Read)XIO(Command_Being_Processed)XIO(Local_Control.11)GEQ(K50ProL2.Command,45)LEQ(K50ProL2.Command,49)OTL(Command_Being_Processed)SUB(K50ProL2.Command,44,CC_W_Index)BTD(K50ProL2.Write_Data.Custom_Color[CC_W_Index].Blue,0,Port_Data.Data_Transfer[0],0,8)BTD(K50ProL2.Write_Data.Custom_Color[CC_W_Index].Green,0,Port_Data.Data_Transfer[1],0,8)BTD(K50ProL2.Write_Data.Custom_Color[CC_W_Index].Red,0,Port_Data.Data_Transfer[2],0,8)CPS(K50ProL2.Write_Data.Custom_Color[CC_W_Index].Color_Name.DATA[0],Port_Data.Data_Transfer[3],8)MOV(Port,Port_Data.Data_Transfer[185])MOV(0,Port_Data.Data_Transfer[187])MOV(65,Port_Data.Data_Transfer[188])MOV(11,Port_Data.Data_Transfer[189])SUB(K50ProL2.Command,42,Inprocess_Index)OTL(Port_Data.Port_Write.[Port])OTL(Local_Control.11);
   44: NOP();
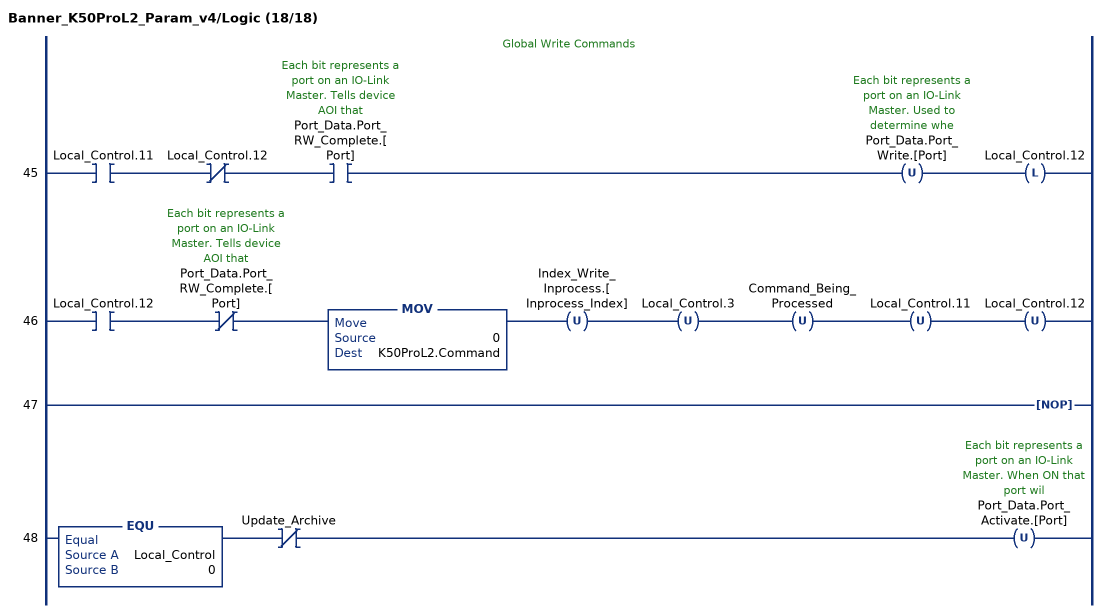
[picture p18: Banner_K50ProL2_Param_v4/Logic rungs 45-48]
   // Global Write Commands
   45: XIC(Local_Control.11)XIO(Local_Control.12)XIC(Port_Data.Port_RW_Complete.[Port])OTU(Port_Data.Port_Write.[Port])OTL(Local_Control.12);
   46: XIC(Local_Control.12)XIO(Port_Data.Port_RW_Complete.[Port])MOV(0,K50ProL2.Command)OTU(Index_Write_Inprocess.[Inprocess_Index])OTU(Local_Control.3)OTU(Command_Being_Processed)OTU(Local_Control.11)OTU(Local_Control.12);
   47: NOP();
   48: EQU(Local_Control,0)XIO(Update_Archive)OTU(Port_Data.Port_Activate.[Port]);
END_ROUTINE
END_ADD_ON_INSTRUCTION
